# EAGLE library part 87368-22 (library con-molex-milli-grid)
RECEPTACAL
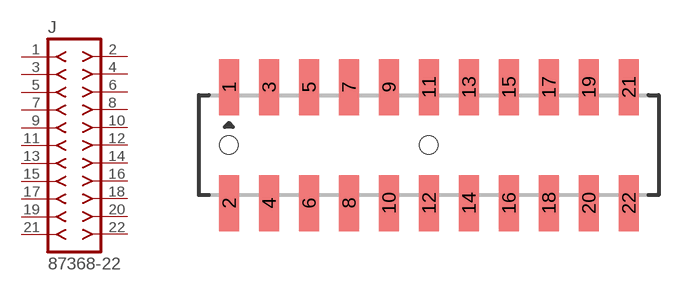
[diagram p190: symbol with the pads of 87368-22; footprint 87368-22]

Designator prefix J

## 87368-22  [87368-22]
1  1  pas
2  2  pas
3  3  pas
4  4  pas
5  5  pas
6  6  pas
7  7  pas
8  8  pas
9  9  pas
10  10  pas
11  11  pas
12  12  pas
13  13  pas
14  14  pas
15  15  pas
16  16  pas
17  17  pas
18  18  pas
19  19  pas
20  20  pas
21  21  pas
22  22  pas

## Footprint 87368-22 (pad centres in mm)
RECEPTACAL SMD Dual Row, Side Entry
smd 1 x 2.8: 1 -10,2.9; 2 -10,-2.9; 3 -8,2.9; 4 -8,-2.9; 5 -6,2.9; 6 -6,-2.9; 7 -4,2.9; 8 -4,-2.9; 9 -2,2.9; 10 -2,-2.9; 11 0,2.9; 12 0,-2.9; 13 2,2.9; 14 2,-2.9; 15 4,2.9; 16 4,-2.9; 17 6,2.9; 18 6,-2.9; 19 8,2.9; 20 8,-2.9; 21 10,2.9; 22 10,-2.9
hole 0.914 at -10,0
hole 0.914 at 0,0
